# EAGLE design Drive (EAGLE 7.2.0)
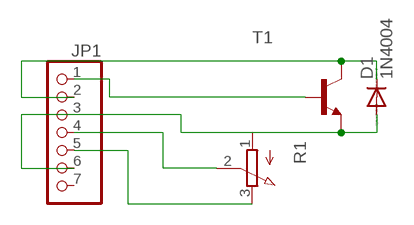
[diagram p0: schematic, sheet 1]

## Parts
D1  1N4004  [DO41-10]
JP1  PINHD-1X7  [1X07]
R1  3RP/1610N  [3RP/1610N]
T1  -NPN-TO220  [TO220]

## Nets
N$1: JP1.1 T1.1(B)
N$2: D1.C JP1.2 T1.2(C)
N$3: D1.A JP1.3 JP1.6 R1.1(A) T1.3(E)
N$4: JP1.5 R1.3(E)
N$5: JP1.4 R1.2(S)
Unconnected: JP1.7

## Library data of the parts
D1 = diode:1N4004: DIODE
JP1 = pinhead:PINHD-1X7: PIN HEADER
R1 = pot:3RP/1610N: 16mm Potentiometer one level Source: http://www.alphapotentiometers.net/html/16mm_pot_2.html
T1 = transistor:*-NPN-: NPN Transistror BF959 corrected 2008.03.06

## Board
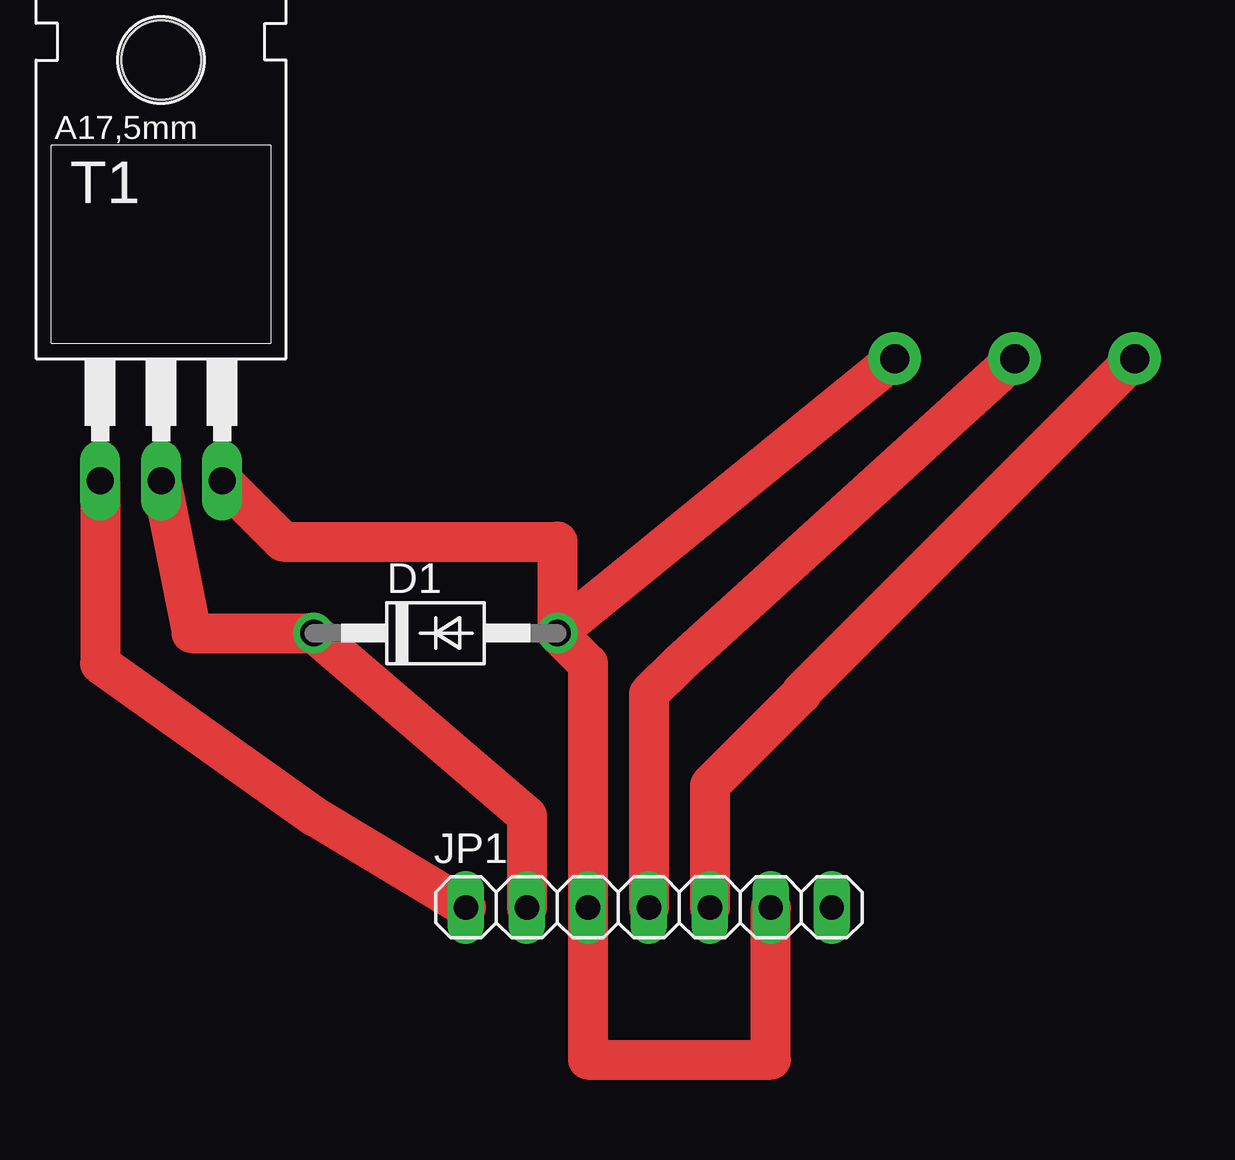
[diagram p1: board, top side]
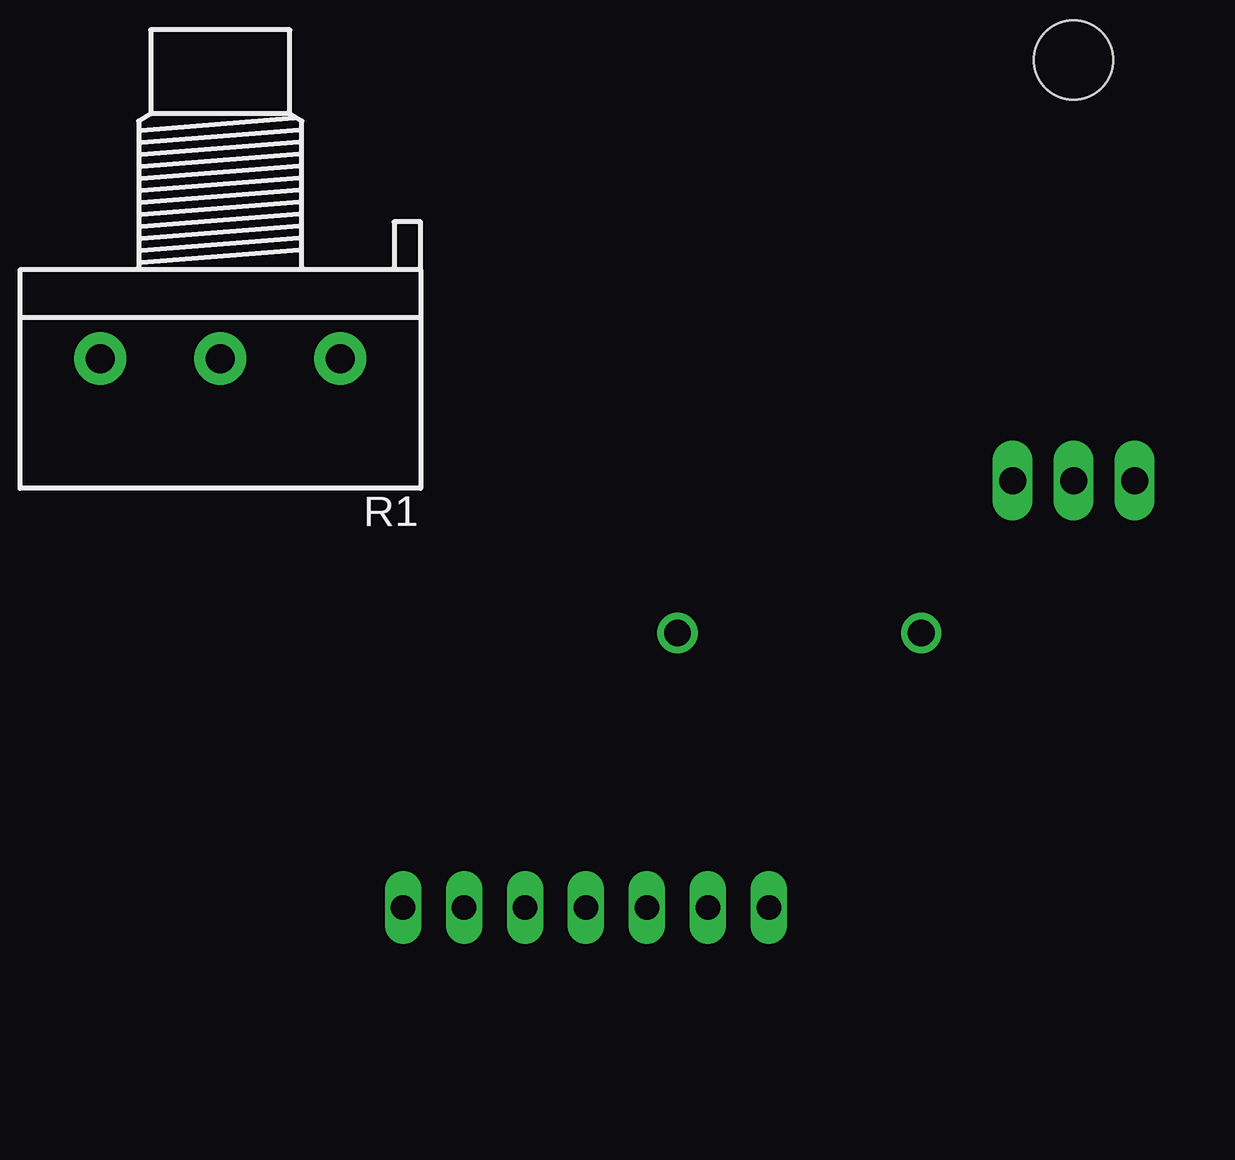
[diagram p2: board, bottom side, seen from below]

No outline drawn. Coordinates in mm, seen from the top.
Copper layers (1*16): Top 0.035mm / dielectric 1.5mm / Bottom 0.035mm
Design rules "default": minimum track width 10mil, minimum drill 24mil, track to track 8mil, track to pad 8mil, pad to pad 8mil, via to via 8mil, smd to smd 8mil, copper to edge 40mil, drill to drill 8mil, minimum pad ring 10mil, minimum via ring 8mil, stop-mask expansion 4mil, vias tented up to drill 0mil, thermal gap 10mil

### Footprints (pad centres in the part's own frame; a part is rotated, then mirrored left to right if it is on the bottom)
DO41-10 = drill 1.118: A 5.08,0; C -5.08,0
1X07 = drill 1.016 long: 1 -7.62,0; 2 -5.08,0; 3 -2.54,0; 4 0,0; 5 2.54,0; 6 5.08,0; 7 7.62,0
3RP/1610N = drill 1.2 pad 2.184: 1 -5,0; 2 0,0; 3 5,0
TO220 = drill 1.118 long: 1 -2.54,-6.35; 2 0,-6.35; 3 2.54,-6.35 | hole 3.302: 0,11.176

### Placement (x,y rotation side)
D1  25.4,17.78 0 top
JP1  34.29,6.35 0 top
R1  49.53,29.21 180 bottom
T1  13.97,30.48 0 top

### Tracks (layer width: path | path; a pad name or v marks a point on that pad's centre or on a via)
N$1
  Top 1.676: T1.1 11.43,16.51 20.32,10.16 JP1.1
N$2
  Top 1.676: T1.2 15.24,17.78 D1.C 29.21,10.16 JP1.2
N$3
  Top 1.676: T1.3 19.05,21.59 30.48,21.59 D1.A | D1.A 31.75,16.51 JP1.3 31.75,0 39.37,0 JP1.6 | R1.1 D1.A
N$4
  Top 1.676: R1.3 40.64,15.32 40.64,15.24 36.83,11.43 JP1.5
N$5
  Top 1.676: R1.2 35.56,16.51 34.29,15.24 JP1.4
